| stm32mp131_133_135 LFBGA289 14x14
[IBIS ver]   4.2
[File name]   stm32mp131_133_135_lfbga289.ibs
[File Rev]   3.4
[Date]   06-03-2024
[Source]   Data Created at STMicroelectronics
[Disclaimer]  This information is for modeling purpose only and is
   not guaranteed.
   The information is subject to change without notice.
[Copyright]   Copyright 2024 STMicroelectronics Inc.
|  You might uncomment [Merged Pins] sections if handeled by the simulation tool
[Component] stm32mp131_133_135_lfbga289
[Manufacturer] STMicroelectronics
[Package]
| variable   typ   min   max
R_pkg  0  NA  NA
L_pkg  0  NA  NA
C_pkg  0  NA  NA
[Pin]   signal_name   model_name
T14  BYPASS_REG1V8  nc
G16  DDR_A0  PDDRIO_PAD
K15  DDR_A1  PDDRIO_PAD
J14  DDR_A10  PDDRIO_PAD
K13  DDR_A11  PDDRIO_PAD
K17  DDR_A12  PDDRIO_PAD
F14  DDR_A13  PDDRIO_PAD
L17  DDR_A14  PDDRIO_PAD
K16  DDR_A15  PDDRIO_PAD
F17  DDR_A2  PDDRIO_PAD
G15  DDR_A3  PDDRIO_PAD
M14  DDR_A4  PDDRIO_PAD
E16  DDR_A5  PDDRIO_PAD
M17  DDR_A6  PDDRIO_PAD
G14  DDR_A7  PDDRIO_PAD
L15  DDR_A8  PDDRIO_PAD
F16  DDR_A9  PDDRIO_PAD
L13  DDR_ATO  nc
G17  DDR_BA0  PDDRIO_PAD
L16  DDR_BA1  PDDRIO_PAD
G13  DDR_BA2  PDDRIO_PAD
J15  DDR_CASN  PDDRIO_PAD
K14  DDR_CKE  PDDRIO_PAD
J17  DDR_CLKN  PDDRIO_PAD
J16  DDR_CLKP  PDDRIO_PAD
H16  DDR_CSN  PDDRIO_PAD
B17  DDR_DQ0  PDDRIO_PAD
C15  DDR_DQ1  PDDRIO_PAD
N15  DDR_DQ10  PDDRIO_PAD
P15  DDR_DQ11  PDDRIO_PAD
R15  DDR_DQ12  PDDRIO_PAD
P16  DDR_DQ13  PDDRIO_PAD
T17  DDR_DQ14  PDDRIO_PAD
T16  DDR_DQ15  PDDRIO_PAD
E13  DDR_DQ2  PDDRIO_PAD
D17  DDR_DQ3  PDDRIO_PAD
B16  DDR_DQ4  PDDRIO_PAD
D16  DDR_DQ5  PDDRIO_PAD
E14  DDR_DQ6  PDDRIO_PAD
E15  DDR_DQ7  PDDRIO_PAD
N16  DDR_DQ8  PDDRIO_PAD
P17  DDR_DQ9  PDDRIO_PAD
D15  DDR_DQM0  PDDRIO_PAD
N14  DDR_DQM1  PDDRIO_PAD
C16  DDR_DQS0N  PDIFF_PAD
C17  DDR_DQS0P  PDIFF_PAD
R16  DDR_DQS1N  PDIFF_PAD
R17  DDR_DQS1P  PDIFF_PAD
L14  DDR_DTO0  PDDRIO_PAD
M16  DDR_DTO1  PDDRIO_PAD
H15  DDR_ODT  PDDRIO_PAD
H17  DDR_RASN  PDDRIO_PAD
E17  DDR_RESETN  PDDRIO_PAD
M13  DDR_VREF  nc
H13  DDR_WEN  PDDRIO_PAD
N17  DDR_ZQ  nc
N9  NJTRST  io8_ft
U10  NRST  nc
R9  NRST_CORE  nc
U3  PA0  io8_ft
R4  PA1  io8_ft
U15  PA10  io8usb_id_otg20_ft
T2  PA11  io8_ft_i2c
E3  PA12  io8_ft_hslv
P3  PA13  io8_ft
T12  PA14  io8_ft
E6  PA15  io8_ft_hslv
P5  PA2  io8_ft
N8  PA3  io8_ft_hslv
U5  PA4  io8_ft
U4  PA5  io8_ft
T8  PA6  io8_ft_hslv
U2  PA7  io8_ft_hslv
M2  PA8  io8_ft_i2c_hslv
A2  PA9  io8_ft_hslv
U7  PB0  io8_ft
T7  PB1  io8_ft_hslv
D10  PB10  io8_ft_hslv
N5  PB11  io8_ft_hslv_et
D9  PB12  io8_ft_hslv
E10  PB13  io8_ft_i2c_hslv
A13  PB14  io8_ft_hslv
B12  PB15  io8_ft_hslv
H4  PB2  io8_ft_hslv
C11  PB3  io8_ft_hslv
B13  PB4  io8_ft_hslv
C10  PB5  io8_ft_hslv
C1  PB6  io8_ft_hslv
A4  PB7  io8_ft_i2c
D1  PB8  io8_ft_i2c
A12  PB9  io8_ft_i2c_hslv
T3  PC0  io8_ft_hslv
U8  PC1  io8_ft_hslv_et
B14  PC10  io8_ft_i2c_hslv
C14  PC11  io8_ft_i2c_hslv
B15  PC12  io8_ft_hslv
K4  PC13  io8_ft
K1  PC14  io8_ft
K2  PC15  io8_ft
U9  PC2  io8_ft_hslv_et
T5  PC3  io8_ft_hslv
U6  PC4  io8_ft
R7  PC5  io8_ft
B11  PC6  io8_ft_hslv
A11  PC7  io8_ft_hslv
D14  PC8  io8_ft_hslv
A16  PC9  io8_ft_hslv
E4  PD0  io8_ft
D5  PD1  io8_ft_i2c_hslv
A3  PD10  io8_ft_hslv
E2  PD11  io8_ft_hslv
C6  PD12  io8_ft_i2c
J1  PD13  io8_ft_hslv
B3  PD14  io8_ft_i2c_hslv
C7  PD15  io8_ft_hslv
A15  PD2  io8_ft_hslv
B1  PD3  io8_ft_i2c
E7  PD4  io8_ft_hslv
A6  PD5  io8_ft_hslv
D2  PD6  io8_ft
N3  PD7  io8_ft_i2c_hslv
C5  PD8  io8_ft
E8  PD9  io8_ft_hslv
T10  PDR_ON  nc
D6  PE0  io8_ft_hslv
B5  PE1  io8_ft_hslv
B8  PE10  io8_ft
D4  PE11  io8_ft_hslv_et
B4  PE12  io8_ft_hslv
C4  PE13  io8_ft_i2c_hslv
C3  PE14  io8_ft_hslv
D8  PE15  io8_ft_i2c_hslv
L1  PE2  io8_ft_i2c_hslv
D13  PE3  io8_ft_hslv
H5  PE4  io8_ft_hslv
T9  PE5  io8_ft_hslv_et
N1  PE6  io8_ft_hslv_et
A5  PE7  io8_ft_hslv
A7  PE8  io8_ft_i2c
B6  PE9  io8_ft_hslv
C13  PF0  io8_ft_hslv
B9  PF1  io8_ft_i2c_hslv
G3  PF10  io8_ft_hslv
T6  PF11  io8_ft
T4  PF12  io8_ft_hslv_et
N6  PF13  io8_ft
P4  PF14  io8_ft
R10  PF15  io8_ft
E9  PF2  io8_ft_i2c_hslv
B10  PF3  io8_ft_i2c_hslv
L2  PF4  io8_ft_hslv
B2  PF5  io8_ft_hslv
G2  PF6  io8_ft_hslv_et
M1  PF7  io8_ft_hslv_et
G5  PF8  io8_ft_hslv
G1  PF9  io8_ft_hslv
D7  PG0  io8_ft_hslv
N2  PG1  io8_ft_hslv_et
F1  PG10  io8_ft_hslv
M3  PG11  io8_ft_hslv_et
T1  PG12  io8_ft
P8  PG13  io8_ft_hslv_et
P9  PG14  io8_ft_hslv_et
G4  PG15  io8_ft_hslv
R1  PG2  io8_ft
L5  PG3  io8_ft_et_i2c_hslv
A8  PG4  io8_ft_hslv
F2  PG5  io8_ft_hslv
A14  PG6  io8_ft_hslv
C9  PG7  io8_ft_hslv
F3  PG8  io8_ft_hslv
E1  PG9  io8_ft_i2c
P1  PH0  io8_ft
P2  PH1  io8_ft
E11  PH10  io8_ft_hslv
H1  PH11  io8_ft_i2c_hslv
C2  PH12  io8_ft_i2c_hslv
A10  PH13  io8_ft_i2c_hslv
B7  PH14  io8_ft_i2c_hslv
F4  PH2  io8_ft_hslv
R2  PH3  io8_ft_i2c_hslv
T15  PH4  io8_ft
R14  PH5  io8_ft
L3  PH6  io8_ft_i2c_hslv
H3  PH7  io8_ft_i2c_hslv
F5  PH8  io8_ft_i2c_hslv
A9  PH9  io8_ft_hslv
L4  PI0  io8_ft
K5  PI1  io8_ft
J3  PI2  io8_ft
H2  PI3  io8_ft
U14  PI4  io8_ft
P12  PI5  io8_ft
R12  PI6  io8_ft
U16  PI7  io8usb_vbus_otg20_ft
R3  PWR_CPU_ON  io8_ft
N13  PWR_LP  io8_ft
P14  PWR_ON  io8_ft
U13  USB_DM1  nc
U11  USB_DM2  nc
T13  USB_DP1  nc
T11  USB_DP2  nc
U12  USB_RREF  nc
J2  VBAT  power
G6  VDD  power
K6  VDD  power
L6  VDD  power
M6  VDD  power
M7  VDD  power
M8  VDD  power
M9  VDD  power
M10  VDD  power
M4  VDD_ANA  power
H8  VDD_CORE  power
H9  VDD_CORE  power
H10  VDD_CORE  power
J8  VDD_CORE  power
J10  VDD_CORE  power
K8  VDD_CORE  power
K9  VDD_CORE  power
K10  VDD_CORE  power
J13  VDD_CORE-J13  power
F6  VDD_CPU  power
F8  VDD_CPU  power
F9  VDD_CPU  power
H6  VDD_CPU  power
J6  VDD_CPU  power
G12  VDD_DDR  power
H12  VDD_DDR  power
J12  VDD_DDR  power
K12  VDD_DDR  power
L12  VDD_DDR  power
M12  VDD_DDR  power
N12  VDD_DDR  power
E12  VDD_DDR-E12-F12  power
F12  VDD_DDR-E12-F12  power
J5  VDD_PLL  power
R13  VDD_PLL2  power
P10  VDD3V3_USBHS  power
P7  VDDA  power
N11  VDDA1V1_REG  power
R11  VDDA1V8_REG  power
F7  VDD-F7-F10-F11  power
F10  VDD-F7-F10-F11  power
F11  VDD-F7-F10-F11  power
M11  VDD-M11  power
C12  VDDSDMMC1  power
D11  VDDSDMMC2  power
P6  VREFN  gnd
R6  VREFP  power
A1  VSS  gnd
A17  VSS  gnd
C8  VSS  gnd
D3  VSS  gnd
D12  VSS  gnd
E5  VSS  gnd
F13  VSS  gnd
F15  VSS  gnd
G7  VSS  gnd
G8  VSS  gnd
G9  VSS  gnd
G10  VSS  gnd
G11  VSS  gnd
H7  VSS  gnd
H11  VSS  gnd
H14  VSS  gnd
J7  VSS  gnd
J9  VSS  gnd
J11  VSS  gnd
K3  VSS  gnd
K7  VSS  gnd
K11  VSS  gnd
L7  VSS  gnd
L8  VSS  gnd
L9  VSS  gnd
L10  VSS  gnd
L11  VSS  gnd
M15  VSS  gnd
N4  VSS  gnd
P11  VSS  gnd
R5  VSS  gnd
R8  VSS  gnd
U1  VSS  gnd
U17  VSS  gnd
M5  VSS_ANA  gnd
J4  VSS_PLL  gnd
P13  VSS_PLL2  gnd
N10  VSS_USBHS  gnd
N7  VSSA  gnd
[Package Model]   501-bga-14x14-289-210615
[Pin Mapping]   pulldown_ref   pullup_ref   | Comment
T14  nc  nc  | Depending on IO usage
| T14  nc  nc  | Depending on IO usage
G16  gnd  vddddr
K15  gnd  vddddr
J14  gnd  vddddr
K13  gnd  vddddr
K17  gnd  vddddr
F14  gnd  vddddr
L17  gnd  vddddr
K16  gnd  vddddr
F17  gnd  vddddr
G15  gnd  vddddr
M14  gnd  vddddr
E16  gnd  vddddr
M17  gnd  vddddr
G14  gnd  vddddr
L15  gnd  vddddr
F16  gnd  vddddr
L13  nc  nc
G17  gnd  vddddr
L16  gnd  vddddr
G13  gnd  vddddr
J15  gnd  vddddr
K14  gnd  vddddr
J17  gnd  vddddr
J16  gnd  vddddr
H16  gnd  vddddr
B17  gnd  vddddr
C15  gnd  vddddr
N15  gnd  vddddr
P15  gnd  vddddr
R15  gnd  vddddr
P16  gnd  vddddr
T17  gnd  vddddr
T16  gnd  vddddr
E13  gnd  vddddr
D17  gnd  vddddr
B16  gnd  vddddr
D16  gnd  vddddr
E14  gnd  vddddr
E15  gnd  vddddr
N16  gnd  vddddr
P17  gnd  vddddr
D15  gnd  vddddr
N14  gnd  vddddr
C16  gnd  vddddr
C17  gnd  vddddr
R16  gnd  vddddr
R17  gnd  vddddr
L14  gnd  vddddr
M16  gnd  vddddr
H15  gnd  vddddr
H17  gnd  vddddr
E17  gnd  vddddr
M13  nc  nc
H13  gnd  vddddr
N17  nc  nc
N9  gnd  vddio
U10  nc  nc
R9  nc  nc
U3  gnd  vddio
R4  gnd  vddio
U15  gnd  vddio
T2  gnd  vddio
E3  gnd  vddio
P3  gnd  vddio
T12  gnd  vddio
E6  gnd  vddio
P5  gnd  vddio
N8  gnd  vddio
U5  gnd  vddio
U4  gnd  vddio
T8  gnd  vddio
U2  gnd  vddio
M2  gnd  vddio
A2  gnd  vddio
U7  gnd  vddio
T7  gnd  vddio
D10  gnd  vddio
N5  gnd  vddio
D9  gnd  vddio
E10  gnd  vddio
A13  gnd  vdds2  | Depending on IO usage
| A13  gnd  vddio  | Depending on IO usage
B12  gnd  vdds2  | Depending on IO usage
| B12  gnd  vddio  | Depending on IO usage
H4  gnd  vddio
C11  gnd  vdds2  | Depending on IO usage
| C11  gnd  vddio  | Depending on IO usage
B13  gnd  vdds2  | Depending on IO usage
| B13  gnd  vddio  | Depending on IO usage
C10  gnd  vddio
C1  gnd  vddio
A4  gnd  vddio
D1  gnd  vddio
A12  gnd  vddio
T3  gnd  vddio
U8  gnd  vddio
B14  gnd  vdds1  | Depending on IO usage
| B14  gnd  vddio  | Depending on IO usage
C14  gnd  vdds1  | Depending on IO usage
| C14  gnd  vddio  | Depending on IO usage
B15  gnd  vdds1  | Depending on IO usage
| B15  gnd  vddio  | Depending on IO usage
K4  gnd  vddio  | Depending on IO usage
| K4  gnd  vbat  | Depending on IO usage
K1  gnd  vddio  | Depending on IO usage
| K1  gnd  vbat  | Depending on IO usage
K2  gnd  vddio  | Depending on IO usage
| K2  gnd  vbat  | Depending on IO usage
U9  gnd  vddio
T5  gnd  vddio
U6  gnd  vddio
R7  gnd  vddio
B11  gnd  vddio
A11  gnd  vddio
D14  gnd  vdds1  | Depending on IO usage
| D14  gnd  vddio  | Depending on IO usage
A16  gnd  vdds1  | Depending on IO usage
| A16  gnd  vddio  | Depending on IO usage
E4  gnd  vddio
D5  gnd  vddio
A3  gnd  vddio
E2  gnd  vddio
C6  gnd  vddio
J1  gnd  vddio
B3  gnd  vddio
C7  gnd  vddio
A15  gnd  vdds1  | Depending on IO usage
| A15  gnd  vddio  | Depending on IO usage
B1  gnd  vddio
E7  gnd  vddio
A6  gnd  vddio
D2  gnd  vddio
N3  gnd  vddio
C5  gnd  vddio
E8  gnd  vddio
T10  nc  nc
D6  gnd  vddio
B5  gnd  vddio
B8  gnd  vddio
D4  gnd  vddio
B4  gnd  vddio
C4  gnd  vddio
C3  gnd  vddio
D8  gnd  vddio
L1  gnd  vddio
D13  gnd  vdds2  | Depending on IO usage
| D13  gnd  vddio  | Depending on IO usage
H5  gnd  vddio
T9  gnd  vddio
N1  gnd  vddio
A5  gnd  vddio
A7  gnd  vddio
B6  gnd  vddio
C13  gnd  vddio
B9  gnd  vddio
G3  gnd  vddio
T6  gnd  vddio
T4  gnd  vddio
N6  gnd  vddio
P4  gnd  vddio
R10  gnd  vddio
E9  gnd  vddio
B10  gnd  vddio
L2  gnd  vddio
B2  gnd  vddio
G2  gnd  vddio
M1  gnd  vddio
G5  gnd  vddio
G1  gnd  vddio
D7  gnd  vddio
N2  gnd  vddio
F1  gnd  vddio
M3  gnd  vddio
T1  gnd  vddio
P8  gnd  vddio
P9  gnd  vddio
G4  gnd  vddio
R1  gnd  vddio
L5  gnd  vddio
A8  gnd  vddio
F2  gnd  vddio
A14  gnd  vdds2  | Depending on IO usage
| A14  gnd  vddio  | Depending on IO usage
C9  gnd  vddio
F3  gnd  vddio
E1  gnd  vddio
P1  gnd  vddio
P2  gnd  vddio
E11  gnd  vddio
H1  gnd  vddio
C2  gnd  vddio
A10  gnd  vddio
B7  gnd  vddio
F4  gnd  vddio
R2  gnd  vddio
T15  gnd  vddio
R14  gnd  vddio
L3  gnd  vddio
H3  gnd  vddio
F5  gnd  vddio
A9  gnd  vddio
L4  gnd  vddio
K5  gnd  vddio  | Depending on IO usage
| K5  gnd  vbat  | Depending on IO usage
J3  gnd  vddio  | Depending on IO usage
| J3  gnd  vbat  | Depending on IO usage
H2  gnd  vddio  | Depending on IO usage
| H2  gnd  vbat  | Depending on IO usage
U14  gnd  vddio
P12  gnd  vddio
R12  gnd  vddio
U16  gnd  vddio
R3  gnd  vddio
N13  gnd  vddio
P14  gnd  vddio
U13  nc  nc  | Depending on IO usage
| U13  nc  nc  | Depending on IO usage
U11  nc  nc  | Depending on IO usage
| U11  nc  nc  | Depending on IO usage
T13  nc  nc  | Depending on IO usage
| T13  nc  nc  | Depending on IO usage
T11  nc  nc  | Depending on IO usage
| T11  nc  nc  | Depending on IO usage
U12  nc  nc  | Depending on IO usage
| U12  nc  nc  | Depending on IO usage
J2  nc  vbat
G6  nc  vddio
K6  nc  vddio
L6  nc  vddio
M6  nc  vddio
M7  nc  vddio
M8  nc  vddio
M9  nc  vddio
M10  nc  vddio
M4  nc  vddana
H8  nc  vddio  | Depending on IO usage
| H8  nc  vbat  | Depending on IO usage
H9  nc  vddio  | Depending on IO usage
| H9  nc  vbat  | Depending on IO usage
H10  nc  vddio  | Depending on IO usage
| H10  nc  vbat  | Depending on IO usage
J8  nc  vddio  | Depending on IO usage
| J8  nc  vbat  | Depending on IO usage
J10  nc  vddio  | Depending on IO usage
| J10  nc  vbat  | Depending on IO usage
K8  nc  vddio  | Depending on IO usage
| K8  nc  vbat  | Depending on IO usage
K9  nc  vddio  | Depending on IO usage
| K9  nc  vbat  | Depending on IO usage
K10  nc  vddio  | Depending on IO usage
| K10  nc  vbat  | Depending on IO usage
J13  nc  vddcore  | Depending on IO usage
| J13  nc  vbat  | Depending on IO usage
F6  nc  vddcpu
F8  nc  vddcpu
F9  nc  vddcpu
H6  nc  vddcpu
J6  nc  vddcpu
G12  nc  vddddr
H12  nc  vddddr
J12  nc  vddddr
K12  nc  vddddr
L12  nc  vddddr
M12  nc  vddddr
N12  nc  vddddr
E12  nc  vddddr
F12  nc  vddddr
J5  nc  vddpll
R13  nc  vddpll2
P10  nc  vdd3v3usbhs
P7  nc  vdda
N11  nc  vdda1v1
R11  nc  vdda1v8
F7  nc  vddio
F10  nc  vddio
F11  nc  vddio
M11  nc  vddio
C12  nc  vdds1
D11  nc  vdds2
P6  gnd  nc
R6  nc  vddio
A1  gnd  nc
A17  gnd  nc
C8  gnd  nc
D3  gnd  nc
D12  gnd  nc
E5  gnd  nc
F13  gnd  nc
F15  gnd  nc
G7  gnd  nc
G8  gnd  nc
G9  gnd  nc
G10  gnd  nc
G11  gnd  nc
H7  gnd  nc
H11  gnd  nc
H14  gnd  nc
J7  gnd  nc
J9  gnd  nc
J11  gnd  nc
K3  gnd  nc
K7  gnd  nc
K11  gnd  nc
L7  gnd  nc
L8  gnd  nc
L9  gnd  nc
L10  gnd  nc
L11  gnd  nc
M15  gnd  nc
N4  gnd  nc
P11  gnd  nc
R5  gnd  nc
R8  gnd  nc
U1  gnd  nc
U17  gnd  nc
M5  gnd  nc
J4  gnd  nc
P13  gnd  nc
N10  gnd  nc
N7  gnd  nc
[Diff_pin]   inv_pin   vdiff   tdelay_typ   tdelay_min   tdelay_max
J16   J17   0.320V   0ns   NA   NA   |CK
C17   C16   0.320V   0ns   NA   NA   |DQS0
R17   R16   0.320V   0ns   NA   NA   |DQS1
[Model Selector] PDIFF_PAD
MSD_D3RF2_18   DDR2 MSD_D3R_PDIFF Z0=18-Ohm
MSD_D3RF2_40   DDR2 MSD_D3R_PDIFF Z0=40-Ohm
MSD_D3RF2_48   DDR2 MSD_D3R_PDIFF Z0=48-Ohm
MSD_D3RF2_ODT150   DDR2 MSD_D3R_PDIFF cell 150-Ohm ODT Receiver
MSD_D3RF2_ODT50   DDR2 MSD_D3R_PDIFF cell 50-Ohm ODT Receiver
MSD_D3RF2_ODT75   DDR2 MSD_D3R_PDIFF cell 75-Ohm ODT Receiver
MSD_D3RF2_ODTOFF   DDR2 MSD_D3R_PDIFF cell ODT off Receiver
MSD_D3RF3_34   DDR3 MSD_D3R_PDIFF cell  Z0=34-Ohm
MSD_D3RF3_40   DDR3 MSD_D3R_PDIFF cell  Z0=40-Ohm
MSD_D3RF3_48   DDR3 MSD_D3R_PDIFF cell  Z0=48-Ohm
MSD_D3RF3L_34   DDR3L MSD_D3R_PDIFF cell  Z0=34-Ohm
MSD_D3RF3L_40   DDR3L MSD_D3R_PDIFF cell  Z0=40-Ohm
MSD_D3RF3L_48   DDR3L MSD_D3R_PDIFF cell  Z0=48-Ohm
MSD_D3RF3L_ODT120   DDR3L MSD_D3R_PDIFF cell 120-Ohm ODT Receiver
MSD_D3RF3L_ODT40   DDR3L MSD_D3R_PDIFF cell 40-Ohm ODT Receiver
MSD_D3RF3L_ODT60   DDR3L MSD_D3R_PDIFF cell 60-Ohm ODT Receiver
MSD_D3RF3L_ODTOFF   DDR3L MSD_D3R_PDIFF cell ODT off Receiver
MSD_D3RF3_ODT120   DDR3 MSD_D3R_PDIFF cell 120-Ohm ODT Receiver
MSD_D3RF3_ODT40   DDR3 MSD_D3R_PDIFF cell 40-Ohm ODT Receiver
MSD_D3RF3_ODT60   DDR3 MSD_D3R_PDIFF cell 60-Ohm ODT Receiver
MSD_D3RF3_ODTOFF   DDR3 MSD_D3R_PDIFF cell ODT off Receiver
MSD_D3RFL2_34   LPDDR2 MSD_D3R_PDIFF cell  Z0=34-Ohm
MSD_D3RFL2_40   LPDDR2 MSD_D3R_PDIFF cell  Z0=40-Ohm
MSD_D3RFL2_48   LPDDR2 MSD_D3R_PDIFF cell  Z0=48-Ohm
MSD_D3RFL2_60   LPDDR2 MSD_D3R_PDIFF cell  Z0=60-Ohm
MSD_D3RFL2_80   LPDDR2 MSD_D3R_PDIFF cell  Z0=80-Ohm
MSD_D3RFL2_ODTOFF   LPDDR2 MSD_D3R_PDIFF cell ODT off Receiver
MSD_D3RFL_48   LPDDR MSD_D3R_PDIFF cell  Z0=48-Ohm
MSD_D3RFL_ODTOFF   LPDDR MSD_D3R_PDIFF cell ODT off Receiver
MSD_D3RF2_18_OPEN   DDR2 MSD_D3R_PDIFF_PDQSR Z0=18-Ohm
MSD_D3RF2_40_OPEN   DDR2 MSD_D3R_PDIFF_PDQSR Z0=40-Ohm
MSD_D3RF2_48_OPEN   DDR2 MSD_D3R_PDIFF_PDQSR Z0=48-Ohm
MSD_D3RF2_18_PD344   DDR2 MSD_D3R_PDIFF_PDQSR Z0=18-Ohm
MSD_D3RF2_40_PD344   DDR2 MSD_D3R_PDIFF_PDQSR Z0=40-Ohm
MSD_D3RF2_48_PD344   DDR2 MSD_D3R_PDIFF_PDQSR Z0=48-Ohm
MSD_D3RF2_18_PD393   DDR2 MSD_D3R_PDIFF_PDQSR Z0=18-Ohm
MSD_D3RF2_40_PD393   DDR2 MSD_D3R_PDIFF_PDQSR Z0=40-Ohm
MSD_D3RF2_48_PD393   DDR2 MSD_D3R_PDIFF_PDQSR Z0=48-Ohm
MSD_D3RF2_18_PD458   DDR2 MSD_D3R_PDIFF_PDQSR Z0=18-Ohm
MSD_D3RF2_40_PD458   DDR2 MSD_D3R_PDIFF_PDQSR Z0=40-Ohm
MSD_D3RF2_48_PD458   DDR2 MSD_D3R_PDIFF_PDQSR Z0=48-Ohm
MSD_D3RF2_18_PD500   DDR2 MSD_D3R_PDIFF_PDQSR Z0=18-Ohm
MSD_D3RF2_40_PD500   DDR2 MSD_D3R_PDIFF_PDQSR Z0=40-Ohm
MSD_D3RF2_48_PD500   DDR2 MSD_D3R_PDIFF_PDQSR Z0=48-Ohm
MSD_D3RF2_18_PD550   DDR2 MSD_D3R_PDIFF_PDQSR Z0=18-Ohm
MSD_D3RF2_40_PD550   DDR2 MSD_D3R_PDIFF_PDQSR Z0=40-Ohm
MSD_D3RF2_48_PD550   DDR2 MSD_D3R_PDIFF_PDQSR Z0=48-Ohm
MSD_D3RF2_18_PD611   DDR2 MSD_D3R_PDIFF_PDQSR Z0=18-Ohm
MSD_D3RF2_40_PD611   DDR2 MSD_D3R_PDIFF_PDQSR Z0=40-Ohm
MSD_D3RF2_48_PD611   DDR2 MSD_D3R_PDIFF_PDQSR Z0=48-Ohm
MSD_D3RF2_18_PD688   DDR2 MSD_D3R_PDIFF_PDQSR Z0=18-Ohm
MSD_D3RF2_40_PD688   DDR2 MSD_D3R_PDIFF_PDQSR Z0=40-Ohm
MSD_D3RF2_48_PD688   DDR2 MSD_D3R_PDIFF_PDQSR Z0=48-Ohm
MSD_D3RF2_18_PU344   DDR2 MSD_D3R_PDIFF_PDQSR Z0=18-Ohm
MSD_D3RF2_40_PU344   DDR2 MSD_D3R_PDIFF_PDQSR Z0=40-Ohm
MSD_D3RF2_48_PU344   DDR2 MSD_D3R_PDIFF_PDQSR Z0=48-Ohm
MSD_D3RF2_18_PU393   DDR2 MSD_D3R_PDIFF_PDQSR Z0=18-Ohm
MSD_D3RF2_40_PU393   DDR2 MSD_D3R_PDIFF_PDQSR Z0=40-Ohm
MSD_D3RF2_48_PU393   DDR2 MSD_D3R_PDIFF_PDQSR Z0=48-Ohm
MSD_D3RF2_18_PU458   DDR2 MSD_D3R_PDIFF_PDQSR Z0=18-Ohm
MSD_D3RF2_40_PU458   DDR2 MSD_D3R_PDIFF_PDQSR Z0=40-Ohm
MSD_D3RF2_48_PU458   DDR2 MSD_D3R_PDIFF_PDQSR Z0=48-Ohm
MSD_D3RF2_18_PU500   DDR2 MSD_D3R_PDIFF_PDQSR Z0=18-Ohm
MSD_D3RF2_40_PU500   DDR2 MSD_D3R_PDIFF_PDQSR Z0=40-Ohm
MSD_D3RF2_48_PU500   DDR2 MSD_D3R_PDIFF_PDQSR Z0=48-Ohm
MSD_D3RF2_18_PU550   DDR2 MSD_D3R_PDIFF_PDQSR Z0=18-Ohm
MSD_D3RF2_40_PU550   DDR2 MSD_D3R_PDIFF_PDQSR Z0=40-Ohm
MSD_D3RF2_48_PU550   DDR2 MSD_D3R_PDIFF_PDQSR Z0=48-Ohm
MSD_D3RF2_18_PU611   DDR2 MSD_D3R_PDIFF_PDQSR Z0=18-Ohm
MSD_D3RF2_40_PU611   DDR2 MSD_D3R_PDIFF_PDQSR Z0=40-Ohm
MSD_D3RF2_48_PU611   DDR2 MSD_D3R_PDIFF_PDQSR Z0=48-Ohm
MSD_D3RF2_18_PU688   DDR2 MSD_D3R_PDIFF_PDQSR Z0=18-Ohm
MSD_D3RF2_40_PU688   DDR2 MSD_D3R_PDIFF_PDQSR Z0=40-Ohm
MSD_D3RF2_48_PU688   DDR2 MSD_D3R_PDIFF_PDQSR Z0=48-Ohm
MSD_D3RF2_18_PWRDWN   DDR2 MSD_D3R_PDIFF_PDQSR Z0=18-Ohm
MSD_D3RF2_40_PWRDWN   DDR2 MSD_D3R_PDIFF_PDQSR Z0=40-Ohm
MSD_D3RF2_48_PWRDWN   DDR2 MSD_D3R_PDIFF_PDQSR Z0=48-Ohm
MSD_D3RF3_34_OPEN   DDR3 MSD_D3R_PDIFF_PDQSR cell  Z0=34-Ohm
MSD_D3RF3_40_OPEN   DDR3 MSD_D3R_PDIFF_PDQSR cell  Z0=40-Ohm
MSD_D3RF3_48_OPEN   DDR3 MSD_D3R_PDIFF_PDQSR cell  Z0=48-Ohm
MSD_D3RF3_34_PD344   DDR3 MSD_D3R_PDIFF_PDQSR cell  Z0=34-Ohm
MSD_D3RF3_40_PD344   DDR3 MSD_D3R_PDIFF_PDQSR cell  Z0=40-Ohm
MSD_D3RF3_48_PD344   DDR3 MSD_D3R_PDIFF_PDQSR cell  Z0=48-Ohm
MSD_D3RF3_34_PD393   DDR3 MSD_D3R_PDIFF_PDQSR cell  Z0=34-Ohm
MSD_D3RF3_40_PD393   DDR3 MSD_D3R_PDIFF_PDQSR cell  Z0=40-Ohm
MSD_D3RF3_48_PD393   DDR3 MSD_D3R_PDIFF_PDQSR cell  Z0=48-Ohm
MSD_D3RF3_34_PD458   DDR3 MSD_D3R_PDIFF_PDQSR cell  Z0=34-Ohm
MSD_D3RF3_40_PD458   DDR3 MSD_D3R_PDIFF_PDQSR cell  Z0=40-Ohm
MSD_D3RF3_48_PD458   DDR3 MSD_D3R_PDIFF_PDQSR cell  Z0=48-Ohm
MSD_D3RF3_34_PD500   DDR3 MSD_D3R_PDIFF_PDQSR cell  Z0=34-Ohm
MSD_D3RF3_40_PD500   DDR3 MSD_D3R_PDIFF_PDQSR cell  Z0=40-Ohm
MSD_D3RF3_48_PD500   DDR3 MSD_D3R_PDIFF_PDQSR cell  Z0=48-Ohm
MSD_D3RF3_34_PD550   DDR3 MSD_D3R_PDIFF_PDQSR cell  Z0=34-Ohm
MSD_D3RF3_40_PD550   DDR3 MSD_D3R_PDIFF_PDQSR cell  Z0=40-Ohm
MSD_D3RF3_48_PD550   DDR3 MSD_D3R_PDIFF_PDQSR cell  Z0=48-Ohm
MSD_D3RF3_34_PD611   DDR3 MSD_D3R_PDIFF_PDQSR cell  Z0=34-Ohm
MSD_D3RF3_40_PD611   DDR3 MSD_D3R_PDIFF_PDQSR cell  Z0=40-Ohm
MSD_D3RF3_48_PD611   DDR3 MSD_D3R_PDIFF_PDQSR cell  Z0=48-Ohm
MSD_D3RF3_34_PD688   DDR3 MSD_D3R_PDIFF_PDQSR cell  Z0=34-Ohm
MSD_D3RF3_40_PD688   DDR3 MSD_D3R_PDIFF_PDQSR cell  Z0=40-Ohm
MSD_D3RF3_48_PD688   DDR3 MSD_D3R_PDIFF_PDQSR cell  Z0=48-Ohm
MSD_D3RF3_34_PU344   DDR3 MSD_D3R_PDIFF_PDQSR cell  Z0=34-Ohm
MSD_D3RF3_40_PU344   DDR3 MSD_D3R_PDIFF_PDQSR cell  Z0=40-Ohm
MSD_D3RF3_48_PU344   DDR3 MSD_D3R_PDIFF_PDQSR cell  Z0=48-Ohm
MSD_D3RF3_34_PU393   DDR3 MSD_D3R_PDIFF_PDQSR cell  Z0=34-Ohm
MSD_D3RF3_40_PU393   DDR3 MSD_D3R_PDIFF_PDQSR cell  Z0=40-Ohm
MSD_D3RF3_48_PU393   DDR3 MSD_D3R_PDIFF_PDQSR cell  Z0=48-Ohm
MSD_D3RF3_34_PU458   DDR3 MSD_D3R_PDIFF_PDQSR cell  Z0=34-Ohm
MSD_D3RF3_40_PU458   DDR3 MSD_D3R_PDIFF_PDQSR cell  Z0=40-Ohm
MSD_D3RF3_48_PU458   DDR3 MSD_D3R_PDIFF_PDQSR cell  Z0=48-Ohm
MSD_D3RF3_34_PU500   DDR3 MSD_D3R_PDIFF_PDQSR cell  Z0=34-Ohm
MSD_D3RF3_40_PU500   DDR3 MSD_D3R_PDIFF_PDQSR cell  Z0=40-Ohm
MSD_D3RF3_48_PU500   DDR3 MSD_D3R_PDIFF_PDQSR cell  Z0=48-Ohm
MSD_D3RF3_34_PU550   DDR3 MSD_D3R_PDIFF_PDQSR cell  Z0=34-Ohm
MSD_D3RF3_40_PU550   DDR3 MSD_D3R_PDIFF_PDQSR cell  Z0=40-Ohm
MSD_D3RF3_48_PU550   DDR3 MSD_D3R_PDIFF_PDQSR cell  Z0=48-Ohm
MSD_D3RF3_34_PU611   DDR3 MSD_D3R_PDIFF_PDQSR cell  Z0=34-Ohm
MSD_D3RF3_40_PU611   DDR3 MSD_D3R_PDIFF_PDQSR cell  Z0=40-Ohm
MSD_D3RF3_48_PU611   DDR3 MSD_D3R_PDIFF_PDQSR cell  Z0=48-Ohm
MSD_D3RF3_34_PU688   DDR3 MSD_D3R_PDIFF_PDQSR cell  Z0=34-Ohm
MSD_D3RF3_40_PU688   DDR3 MSD_D3R_PDIFF_PDQSR cell  Z0=40-Ohm
MSD_D3RF3_48_PU688   DDR3 MSD_D3R_PDIFF_PDQSR cell  Z0=48-Ohm
MSD_D3RF3_34_PWRDWN   DDR3 MSD_D3R_PDIFF_PDQSR cell  Z0=34-Ohm
MSD_D3RF3_40_PWRDWN   DDR3 MSD_D3R_PDIFF_PDQSR cell  Z0=40-Ohm
MSD_D3RF3_48_PWRDWN   DDR3 MSD_D3R_PDIFF_PDQSR cell  Z0=48-Ohm
MSD_D3RF3L_34_OPEN   DDR3L MSD_D3R_PDIFF_PDQSR cell  Z0=34-Ohm
MSD_D3RF3L_40_OPEN   DDR3L MSD_D3R_PDIFF_PDQSR cell  Z0=40-Ohm
MSD_D3RF3L_48_OPEN   DDR3L MSD_D3R_PDIFF_PDQSR cell  Z0=48-Ohm
MSD_D3RF3L_34_PD344   DDR3L MSD_D3R_PDIFF_PDQSR cell  Z0=34-Ohm
MSD_D3RF3L_40_PD344   DDR3L MSD_D3R_PDIFF_PDQSR cell  Z0=40-Ohm
MSD_D3RF3L_48_PD344   DDR3L MSD_D3R_PDIFF_PDQSR cell  Z0=48-Ohm
MSD_D3RF3L_34_PD393   DDR3L MSD_D3R_PDIFF_PDQSR cell  Z0=34-Ohm
MSD_D3RF3L_40_PD393   DDR3L MSD_D3R_PDIFF_PDQSR cell  Z0=40-Ohm
MSD_D3RF3L_48_PD393   DDR3L MSD_D3R_PDIFF_PDQSR cell  Z0=48-Ohm
MSD_D3RF3L_34_PD458   DDR3L MSD_D3R_PDIFF_PDQSR cell  Z0=34-Ohm
MSD_D3RF3L_40_PD458   DDR3L MSD_D3R_PDIFF_PDQSR cell  Z0=40-Ohm
MSD_D3RF3L_48_PD458   DDR3L MSD_D3R_PDIFF_PDQSR cell  Z0=48-Ohm
MSD_D3RF3L_34_PD500   DDR3L MSD_D3R_PDIFF_PDQSR cell  Z0=34-Ohm
MSD_D3RF3L_40_PD500   DDR3L MSD_D3R_PDIFF_PDQSR cell  Z0=40-Ohm
MSD_D3RF3L_48_PD500   DDR3L MSD_D3R_PDIFF_PDQSR cell  Z0=48-Ohm
MSD_D3RF3L_34_PD550   DDR3L MSD_D3R_PDIFF_PDQSR cell  Z0=34-Ohm
MSD_D3RF3L_40_PD550   DDR3L MSD_D3R_PDIFF_PDQSR cell  Z0=40-Ohm
MSD_D3RF3L_48_PD550   DDR3L MSD_D3R_PDIFF_PDQSR cell  Z0=48-Ohm
MSD_D3RF3L_34_PD611   DDR3L MSD_D3R_PDIFF_PDQSR cell  Z0=34-Ohm
MSD_D3RF3L_40_PD611   DDR3L MSD_D3R_PDIFF_PDQSR cell  Z0=40-Ohm
MSD_D3RF3L_48_PD611   DDR3L MSD_D3R_PDIFF_PDQSR cell  Z0=48-Ohm
MSD_D3RF3L_34_PD688   DDR3L MSD_D3R_PDIFF_PDQSR cell  Z0=34-Ohm
MSD_D3RF3L_40_PD688   DDR3L MSD_D3R_PDIFF_PDQSR cell  Z0=40-Ohm
MSD_D3RF3L_48_PD688   DDR3L MSD_D3R_PDIFF_PDQSR cell  Z0=48-Ohm
MSD_D3RF3L_34_PU344   DDR3L MSD_D3R_PDIFF_PDQSR cell  Z0=34-Ohm
MSD_D3RF3L_40_PU344   DDR3L MSD_D3R_PDIFF_PDQSR cell  Z0=40-Ohm
MSD_D3RF3L_48_PU344   DDR3L MSD_D3R_PDIFF_PDQSR cell  Z0=48-Ohm
MSD_D3RF3L_34_PU393   DDR3L MSD_D3R_PDIFF_PDQSR cell  Z0=34-Ohm
MSD_D3RF3L_40_PU393   DDR3L MSD_D3R_PDIFF_PDQSR cell  Z0=40-Ohm
MSD_D3RF3L_48_PU393   DDR3L MSD_D3R_PDIFF_PDQSR cell  Z0=48-Ohm
MSD_D3RF3L_34_PU458   DDR3L MSD_D3R_PDIFF_PDQSR cell  Z0=34-Ohm
MSD_D3RF3L_40_PU458   DDR3L MSD_D3R_PDIFF_PDQSR cell  Z0=40-Ohm
MSD_D3RF3L_48_PU458   DDR3L MSD_D3R_PDIFF_PDQSR cell  Z0=48-Ohm
MSD_D3RF3L_34_PU500   DDR3L MSD_D3R_PDIFF_PDQSR cell  Z0=34-Ohm
MSD_D3RF3L_40_PU500   DDR3L MSD_D3R_PDIFF_PDQSR cell  Z0=40-Ohm
MSD_D3RF3L_48_PU500   DDR3L MSD_D3R_PDIFF_PDQSR cell  Z0=48-Ohm
MSD_D3RF3L_34_PU550   DDR3L MSD_D3R_PDIFF_PDQSR cell  Z0=34-Ohm
MSD_D3RF3L_40_PU550   DDR3L MSD_D3R_PDIFF_PDQSR cell  Z0=40-Ohm
MSD_D3RF3L_48_PU550   DDR3L MSD_D3R_PDIFF_PDQSR cell  Z0=48-Ohm
MSD_D3RF3L_34_PU611   DDR3L MSD_D3R_PDIFF_PDQSR cell  Z0=34-Ohm
MSD_D3RF3L_40_PU611   DDR3L MSD_D3R_PDIFF_PDQSR cell  Z0=40-Ohm
MSD_D3RF3L_48_PU611   DDR3L MSD_D3R_PDIFF_PDQSR cell  Z0=48-Ohm
MSD_D3RF3L_34_PU688   DDR3L MSD_D3R_PDIFF_PDQSR cell  Z0=34-Ohm
MSD_D3RF3L_40_PU688   DDR3L MSD_D3R_PDIFF_PDQSR cell  Z0=40-Ohm
MSD_D3RF3L_48_PU688   DDR3L MSD_D3R_PDIFF_PDQSR cell  Z0=48-Ohm
MSD_D3RF3L_34_PWRDWN   DDR3L MSD_D3R_PDIFF_PDQSR cell  Z0=34-Ohm
MSD_D3RF3L_40_PWRDWN   DDR3L MSD_D3R_PDIFF_PDQSR cell  Z0=40-Ohm
MSD_D3RF3L_48_PWRDWN   DDR3L MSD_D3R_PDIFF_PDQSR cell  Z0=48-Ohm
MSD_D3RFL2_34_OPEN   LPDDR2 MSD_D3R_PDIFF_PDQSR cell  Z0=34-Ohm
MSD_D3RFL2_40_OPEN   LPDDR2 MSD_D3R_PDIFF_PDQSR cell  Z0=40-Ohm
MSD_D3RFL2_48_OPEN   LPDDR2 MSD_D3R_PDIFF_PDQSR cell  Z0=48-Ohm
MSD_D3RFL2_60_OPEN   LPDDR2 MSD_D3R_PDIFF_PDQSR cell  Z0=60-Ohm
MSD_D3RFL2_80_OPEN   LPDDR2 MSD_D3R_PDIFF_PDQSR cell  Z0=80-Ohm
MSD_D3RFL_48_OPEN   LPDDR MSD_D3R_PDIFF_PDQSR cell  Z0=48-Ohm
MSD_D3RFL2_34_PD344   LPDDR2 MSD_D3R_PDIFF_PDQSR cell  Z0=34-Ohm
MSD_D3RFL2_40_PD344   LPDDR2 MSD_D3R_PDIFF_PDQSR cell  Z0=40-Ohm
MSD_D3RFL2_48_PD344   LPDDR2 MSD_D3R_PDIFF_PDQSR cell  Z0=48-Ohm
MSD_D3RFL2_60_PD344   LPDDR2 MSD_D3R_PDIFF_PDQSR cell  Z0=60-Ohm
MSD_D3RFL2_80_PD344   LPDDR2 MSD_D3R_PDIFF_PDQSR cell  Z0=80-Ohm
MSD_D3RFL_48_PD344   LPDDR MSD_D3R_PDIFF_PDQSR cell  Z0=48-Ohm
MSD_D3RFL2_34_PD393   LPDDR2 MSD_D3R_PDIFF_PDQSR cell  Z0=34-Ohm
MSD_D3RFL2_40_PD393   LPDDR2 MSD_D3R_PDIFF_PDQSR cell  Z0=40-Ohm
MSD_D3RFL2_48_PD393   LPDDR2 MSD_D3R_PDIFF_PDQSR cell  Z0=48-Ohm
MSD_D3RFL2_60_PD393   LPDDR2 MSD_D3R_PDIFF_PDQSR cell  Z0=60-Ohm
MSD_D3RFL2_80_PD393   LPDDR2 MSD_D3R_PDIFF_PDQSR cell  Z0=80-Ohm
MSD_D3RFL_48_PD393   LPDDR MSD_D3R_PDIFF_PDQSR cell  Z0=48-Ohm
MSD_D3RFL2_34_PD458   LPDDR2 MSD_D3R_PDIFF_PDQSR cell  Z0=34-Ohm
MSD_D3RFL2_40_PD458   LPDDR2 MSD_D3R_PDIFF_PDQSR cell  Z0=40-Ohm
MSD_D3RFL2_48_PD458   LPDDR2 MSD_D3R_PDIFF_PDQSR cell  Z0=48-Ohm
MSD_D3RFL2_60_PD458   LPDDR2 MSD_D3R_PDIFF_PDQSR cell  Z0=60-Ohm
MSD_D3RFL2_80_PD458   LPDDR2 MSD_D3R_PDIFF_PDQSR cell  Z0=80-Ohm
MSD_D3RFL_48_PD458   LPDDR MSD_D3R_PDIFF_PDQSR cell  Z0=48-Ohm
MSD_D3RFL2_34_PD500   LPDDR2 MSD_D3R_PDIFF_PDQSR cell  Z0=34-Ohm
MSD_D3RFL2_40_PD500   LPDDR2 MSD_D3R_PDIFF_PDQSR cell  Z0=40-Ohm
MSD_D3RFL2_48_PD500   LPDDR2 MSD_D3R_PDIFF_PDQSR cell  Z0=48-Ohm
MSD_D3RFL2_60_PD500   LPDDR2 MSD_D3R_PDIFF_PDQSR cell  Z0=60-Ohm
MSD_D3RFL2_80_PD500   LPDDR2 MSD_D3R_PDIFF_PDQSR cell  Z0=80-Ohm
MSD_D3RFL_48_PD500   LPDDR MSD_D3R_PDIFF_PDQSR cell  Z0=48-Ohm
MSD_D3RFL2_34_PD550   LPDDR2 MSD_D3R_PDIFF_PDQSR cell  Z0=34-Ohm
MSD_D3RFL2_40_PD550   LPDDR2 MSD_D3R_PDIFF_PDQSR cell  Z0=40-Ohm
MSD_D3RFL2_48_PD550   LPDDR2 MSD_D3R_PDIFF_PDQSR cell  Z0=48-Ohm
MSD_D3RFL2_60_PD550   LPDDR2 MSD_D3R_PDIFF_PDQSR cell  Z0=60-Ohm
MSD_D3RFL2_80_PD550   LPDDR2 MSD_D3R_PDIFF_PDQSR cell  Z0=80-Ohm
MSD_D3RFL_48_PD550   LPDDR MSD_D3R_PDIFF_PDQSR cell  Z0=48-Ohm
MSD_D3RFL2_34_PD611   LPDDR2 MSD_D3R_PDIFF_PDQSR cell  Z0=34-Ohm
MSD_D3RFL2_40_PD611   LPDDR2 MSD_D3R_PDIFF_PDQSR cell  Z0=40-Ohm
MSD_D3RFL2_48_PD611   LPDDR2 MSD_D3R_PDIFF_PDQSR cell  Z0=48-Ohm
MSD_D3RFL2_60_PD611   LPDDR2 MSD_D3R_PDIFF_PDQSR cell  Z0=60-Ohm
MSD_D3RFL2_80_PD611   LPDDR2 MSD_D3R_PDIFF_PDQSR cell  Z0=80-Ohm
MSD_D3RFL_48_PD611   LPDDR MSD_D3R_PDIFF_PDQSR cell  Z0=48-Ohm
MSD_D3RFL2_34_PD688   LPDDR2 MSD_D3R_PDIFF_PDQSR cell  Z0=34-Ohm
MSD_D3RFL2_40_PD688   LPDDR2 MSD_D3R_PDIFF_PDQSR cell  Z0=40-Ohm
MSD_D3RFL2_48_PD688   LPDDR2 MSD_D3R_PDIFF_PDQSR cell  Z0=48-Ohm
MSD_D3RFL2_60_PD688   LPDDR2 MSD_D3R_PDIFF_PDQSR cell  Z0=60-Ohm
MSD_D3RFL2_80_PD688   LPDDR2 MSD_D3R_PDIFF_PDQSR cell  Z0=80-Ohm
MSD_D3RFL_48_PD688   LPDDR MSD_D3R_PDIFF_PDQSR cell  Z0=48-Ohm
MSD_D3RFL2_34_PU344   LPDDR2 MSD_D3R_PDIFF_PDQSR cell  Z0=34-Ohm
MSD_D3RFL2_40_PU344   LPDDR2 MSD_D3R_PDIFF_PDQSR cell  Z0=40-Ohm
MSD_D3RFL2_48_PU344   LPDDR2 MSD_D3R_PDIFF_PDQSR cell  Z0=48-Ohm
MSD_D3RFL2_60_PU344   LPDDR2 MSD_D3R_PDIFF_PDQSR cell  Z0=60-Ohm
MSD_D3RFL2_80_PU344   LPDDR2 MSD_D3R_PDIFF_PDQSR cell  Z0=80-Ohm
MSD_D3RFL_48_PU344   LPDDR MSD_D3R_PDIFF_PDQSR cell  Z0=48-Ohm
MSD_D3RFL2_34_PU393   LPDDR2 MSD_D3R_PDIFF_PDQSR cell  Z0=34-Ohm
MSD_D3RFL2_40_PU393   LPDDR2 MSD_D3R_PDIFF_PDQSR cell  Z0=40-Ohm
MSD_D3RFL2_48_PU393   LPDDR2 MSD_D3R_PDIFF_PDQSR cell  Z0=48-Ohm
MSD_D3RFL2_60_PU393   LPDDR2 MSD_D3R_PDIFF_PDQSR cell  Z0=60-Ohm
MSD_D3RFL2_80_PU393   LPDDR2 MSD_D3R_PDIFF_PDQSR cell  Z0=80-Ohm
MSD_D3RFL_48_PU393   LPDDR MSD_D3R_PDIFF_PDQSR cell  Z0=48-Ohm
MSD_D3RFL2_34_PU458   LPDDR2 MSD_D3R_PDIFF_PDQSR cell  Z0=34-Ohm
MSD_D3RFL2_40_PU458   LPDDR2 MSD_D3R_PDIFF_PDQSR cell  Z0=40-Ohm
MSD_D3RFL2_48_PU458   LPDDR2 MSD_D3R_PDIFF_PDQSR cell  Z0=48-Ohm
MSD_D3RFL2_60_PU458   LPDDR2 MSD_D3R_PDIFF_PDQSR cell  Z0=60-Ohm
MSD_D3RFL2_80_PU458   LPDDR2 MSD_D3R_PDIFF_PDQSR cell  Z0=80-Ohm
MSD_D3RFL_48_PU458   LPDDR MSD_D3R_PDIFF_PDQSR cell  Z0=48-Ohm
MSD_D3RFL2_34_PU500   LPDDR2 MSD_D3R_PDIFF_PDQSR cell  Z0=34-Ohm
MSD_D3RFL2_40_PU500   LPDDR2 MSD_D3R_PDIFF_PDQSR cell  Z0=40-Ohm
MSD_D3RFL2_48_PU500   LPDDR2 MSD_D3R_PDIFF_PDQSR cell  Z0=48-Ohm
MSD_D3RFL2_60_PU500   LPDDR2 MSD_D3R_PDIFF_PDQSR cell  Z0=60-Ohm
MSD_D3RFL2_80_PU500   LPDDR2 MSD_D3R_PDIFF_PDQSR cell  Z0=80-Ohm
MSD_D3RFL_48_PU500   LPDDR MSD_D3R_PDIFF_PDQSR cell  Z0=48-Ohm
MSD_D3RFL2_34_PU550   LPDDR2 MSD_D3R_PDIFF_PDQSR cell  Z0=34-Ohm
MSD_D3RFL2_40_PU550   LPDDR2 MSD_D3R_PDIFF_PDQSR cell  Z0=40-Ohm
MSD_D3RFL2_48_PU550   LPDDR2 MSD_D3R_PDIFF_PDQSR cell  Z0=48-Ohm
MSD_D3RFL2_60_PU550   LPDDR2 MSD_D3R_PDIFF_PDQSR cell  Z0=60-Ohm
MSD_D3RFL2_80_PU550   LPDDR2 MSD_D3R_PDIFF_PDQSR cell  Z0=80-Ohm
MSD_D3RFL_48_PU550   LPDDR MSD_D3R_PDIFF_PDQSR cell  Z0=48-Ohm
MSD_D3RFL2_34_PU611   LPDDR2 MSD_D3R_PDIFF_PDQSR cell  Z0=34-Ohm
MSD_D3RFL2_40_PU611   LPDDR2 MSD_D3R_PDIFF_PDQSR cell  Z0=40-Ohm
MSD_D3RFL2_48_PU611   LPDDR2 MSD_D3R_PDIFF_PDQSR cell  Z0=48-Ohm
MSD_D3RFL2_60_PU611   LPDDR2 MSD_D3R_PDIFF_PDQSR cell  Z0=60-Ohm
MSD_D3RFL2_80_PU611   LPDDR2 MSD_D3R_PDIFF_PDQSR cell  Z0=80-Ohm
MSD_D3RFL_48_PU611   LPDDR MSD_D3R_PDIFF_PDQSR cell  Z0=48-Ohm
MSD_D3RFL2_34_PU688   LPDDR2 MSD_D3R_PDIFF_PDQSR cell  Z0=34-Ohm
MSD_D3RFL2_40_PU688   LPDDR2 MSD_D3R_PDIFF_PDQSR cell  Z0=40-Ohm
MSD_D3RFL2_48_PU688   LPDDR2 MSD_D3R_PDIFF_PDQSR cell  Z0=48-Ohm
MSD_D3RFL2_60_PU688   LPDDR2 MSD_D3R_PDIFF_PDQSR cell  Z0=60-Ohm
MSD_D3RFL2_80_PU688   LPDDR2 MSD_D3R_PDIFF_PDQSR cell  Z0=80-Ohm
MSD_D3RFL_48_PU688   LPDDR MSD_D3R_PDIFF_PDQSR cell  Z0=48-Ohm
MSD_D3RFL2_34_PWRDWN   LPDDR2 MSD_D3R_PDIFF_PDQSR cell  Z0=34-Ohm
MSD_D3RFL2_40_PWRDWN   LPDDR2 MSD_D3R_PDIFF_PDQSR cell  Z0=40-Ohm
MSD_D3RFL2_48_PWRDWN   LPDDR2 MSD_D3R_PDIFF_PDQSR cell  Z0=48-Ohm
MSD_D3RFL2_60_PWRDWN   LPDDR2 MSD_D3R_PDIFF_PDQSR cell  Z0=60-Ohm
MSD_D3RFL2_80_PWRDWN   LPDDR2 MSD_D3R_PDIFF_PDQSR cell  Z0=80-Ohm
MSD_D3RFL_48_PWRDWN   LPDDR MSD_D3R_PDIFF_PDQSR cell  Z0=48-Ohm
MSD_D3RF2_ODT150_OPEN   DDR2 MSD_D3R_PDIFF_PDQSR cell 150-Ohm ODT Receiver
MSD_D3RF2_ODT50_OPEN   DDR2 MSD_D3R_PDIFF_PDQSR cell 50-Ohm ODT Receiver
MSD_D3RF2_ODT75_OPEN   DDR2 MSD_D3R_PDIFF_PDQSR cell 75-Ohm ODT Receiver
MSD_D3RF2_ODTOFF_OPEN   DDR2 MSD_D3R_PDIFF_PDQSR cell ODT off Receiver
MSD_D3RF2_ODT150_PD344   DDR2 MSD_D3R_PDIFF_PDQSR cell 150-Ohm ODT Receiver
MSD_D3RF2_ODT50_PD344   DDR2 MSD_D3R_PDIFF_PDQSR cell 50-Ohm ODT Receiver
MSD_D3RF2_ODT75_PD344   DDR2 MSD_D3R_PDIFF_PDQSR cell 75-Ohm ODT Receiver
MSD_D3RF2_ODTOFF_PD344   DDR2 MSD_D3R_PDIFF_PDQSR cell ODT off Receiver
MSD_D3RF2_ODT150_PD393   DDR2 MSD_D3R_PDIFF_PDQSR cell 150-Ohm ODT Receiver
MSD_D3RF2_ODT50_PD393   DDR2 MSD_D3R_PDIFF_PDQSR cell 50-Ohm ODT Receiver
MSD_D3RF2_ODT75_PD393   DDR2 MSD_D3R_PDIFF_PDQSR cell 75-Ohm ODT Receiver
MSD_D3RF2_ODTOFF_PD393   DDR2 MSD_D3R_PDIFF_PDQSR cell ODT off Receiver
MSD_D3RF2_ODT150_PD458   DDR2 MSD_D3R_PDIFF_PDQSR cell 150-Ohm ODT Receiver
MSD_D3RF2_ODT50_PD458   DDR2 MSD_D3R_PDIFF_PDQSR cell 50-Ohm ODT Receiver
MSD_D3RF2_ODT75_PD458   DDR2 MSD_D3R_PDIFF_PDQSR cell 75-Ohm ODT Receiver
MSD_D3RF2_ODTOFF_PD458   DDR2 MSD_D3R_PDIFF_PDQSR cell ODT off Receiver
MSD_D3RF2_ODT150_PD500   DDR2 MSD_D3R_PDIFF_PDQSR cell 150-Ohm ODT Receiver
MSD_D3RF2_ODT50_PD500   DDR2 MSD_D3R_PDIFF_PDQSR cell 50-Ohm ODT Receiver
MSD_D3RF2_ODT75_PD500   DDR2 MSD_D3R_PDIFF_PDQSR cell 75-Ohm ODT Receiver
MSD_D3RF2_ODTOFF_PD500   DDR2 MSD_D3R_PDIFF_PDQSR cell ODT off Receiver
MSD_D3RF2_ODT150_PD550   DDR2 MSD_D3R_PDIFF_PDQSR cell 150-Ohm ODT Receiver
MSD_D3RF2_ODT50_PD550   DDR2 MSD_D3R_PDIFF_PDQSR cell 50-Ohm ODT Receiver
MSD_D3RF2_ODT75_PD550   DDR2 MSD_D3R_PDIFF_PDQSR cell 75-Ohm ODT Receiver
MSD_D3RF2_ODTOFF_PD550   DDR2 MSD_D3R_PDIFF_PDQSR cell ODT off Receiver
MSD_D3RF2_ODT150_PD611   DDR2 MSD_D3R_PDIFF_PDQSR cell 150-Ohm ODT Receiver
MSD_D3RF2_ODT50_PD611   DDR2 MSD_D3R_PDIFF_PDQSR cell 50-Ohm ODT Receiver
MSD_D3RF2_ODT75_PD611   DDR2 MSD_D3R_PDIFF_PDQSR cell 75-Ohm ODT Receiver
MSD_D3RF2_ODTOFF_PD611   DDR2 MSD_D3R_PDIFF_PDQSR cell ODT off Receiver
MSD_D3RF2_ODT150_PD688   DDR2 MSD_D3R_PDIFF_PDQSR cell 150-Ohm ODT Receiver
MSD_D3RF2_ODT50_PD688   DDR2 MSD_D3R_PDIFF_PDQSR cell 50-Ohm ODT Receiver
MSD_D3RF2_ODT75_PD688   DDR2 MSD_D3R_PDIFF_PDQSR cell 75-Ohm ODT Receiver
MSD_D3RF2_ODTOFF_PD688   DDR2 MSD_D3R_PDIFF_PDQSR cell ODT off Receiver
MSD_D3RF2_ODT150_PU344   DDR2 MSD_D3R_PDIFF_PDQSR cell 150-Ohm ODT Receiver
MSD_D3RF2_ODT50_PU344   DDR2 MSD_D3R_PDIFF_PDQSR cell 50-Ohm ODT Receiver
MSD_D3RF2_ODT75_PU344   DDR2 MSD_D3R_PDIFF_PDQSR cell 75-Ohm ODT Receiver
MSD_D3RF2_ODTOFF_PU344   DDR2 MSD_D3R_PDIFF_PDQSR cell ODT off Receiver
MSD_D3RF2_ODT150_PU393   DDR2 MSD_D3R_PDIFF_PDQSR cell 150-Ohm ODT Receiver
MSD_D3RF2_ODT50_PU393   DDR2 MSD_D3R_PDIFF_PDQSR cell 50-Ohm ODT Receiver
MSD_D3RF2_ODT75_PU393   DDR2 MSD_D3R_PDIFF_PDQSR cell 75-Ohm ODT Receiver
MSD_D3RF2_ODTOFF_PU393   DDR2 MSD_D3R_PDIFF_PDQSR cell ODT off Receiver
MSD_D3RF2_ODT150_PU458   DDR2 MSD_D3R_PDIFF_PDQSR cell 150-Ohm ODT Receiver
MSD_D3RF2_ODT50_PU458   DDR2 MSD_D3R_PDIFF_PDQSR cell 50-Ohm ODT Receiver
MSD_D3RF2_ODT75_PU458   DDR2 MSD_D3R_PDIFF_PDQSR cell 75-Ohm ODT Receiver
MSD_D3RF2_ODTOFF_PU458   DDR2 MSD_D3R_PDIFF_PDQSR cell ODT off Receiver
MSD_D3RF2_ODT150_PU500   DDR2 MSD_D3R_PDIFF_PDQSR cell 150-Ohm ODT Receiver
MSD_D3RF2_ODT50_PU500   DDR2 MSD_D3R_PDIFF_PDQSR cell 50-Ohm ODT Receiver
MSD_D3RF2_ODT75_PU500   DDR2 MSD_D3R_PDIFF_PDQSR cell 75-Ohm ODT Receiver
MSD_D3RF2_ODTOFF_PU500   DDR2 MSD_D3R_PDIFF_PDQSR cell ODT off Receiver
MSD_D3RF2_ODT150_PU550   DDR2 MSD_D3R_PDIFF_PDQSR cell 150-Ohm ODT Receiver
MSD_D3RF2_ODT50_PU550   DDR2 MSD_D3R_PDIFF_PDQSR cell 50-Ohm ODT Receiver
MSD_D3RF2_ODT75_PU550   DDR2 MSD_D3R_PDIFF_PDQSR cell 75-Ohm ODT Receiver
MSD_D3RF2_ODTOFF_PU550   DDR2 MSD_D3R_PDIFF_PDQSR cell ODT off Receiver
MSD_D3RF2_ODT150_PU611   DDR2 MSD_D3R_PDIFF_PDQSR cell 150-Ohm ODT Receiver
MSD_D3RF2_ODT50_PU611   DDR2 MSD_D3R_PDIFF_PDQSR cell 50-Ohm ODT Receiver
MSD_D3RF2_ODT75_PU611   DDR2 MSD_D3R_PDIFF_PDQSR cell 75-Ohm ODT Receiver
MSD_D3RF2_ODTOFF_PU611   DDR2 MSD_D3R_PDIFF_PDQSR cell ODT off Receiver
MSD_D3RF2_ODT150_PU688   DDR2 MSD_D3R_PDIFF_PDQSR cell 150-Ohm ODT Receiver
MSD_D3RF2_ODT50_PU688   DDR2 MSD_D3R_PDIFF_PDQSR cell 50-Ohm ODT Receiver
MSD_D3RF2_ODT75_PU688   DDR2 MSD_D3R_PDIFF_PDQSR cell 75-Ohm ODT Receiver
MSD_D3RF2_ODTOFF_PU688   DDR2 MSD_D3R_PDIFF_PDQSR cell ODT off Receiver
MSD_D3RF2_ODT150_PWRDWN   DDR2 MSD_D3R_PDIFF_PDQSR cell 150-Ohm ODT Receiver
MSD_D3RF2_ODT50_PWRDWN   DDR2 MSD_D3R_PDIFF_PDQSR cell 50-Ohm ODT Receiver
MSD_D3RF2_ODT75_PWRDWN   DDR2 MSD_D3R_PDIFF_PDQSR cell 75-Ohm ODT Receiver
MSD_D3RF2_ODTOFF_PWRDWN   DDR2 MSD_D3R_PDIFF_PDQSR cell ODT off Receiver
MSD_D3RF3_ODT120_OPEN   DDR3 MSD_D3R_PDIFF_PDQSR cell 120-Ohm ODT Receiver
MSD_D3RF3_ODT40_OPEN   DDR3 MSD_D3R_PDIFF_PDQSR cell 40-Ohm ODT Receiver
MSD_D3RF3_ODT60_OPEN   DDR3 MSD_D3R_PDIFF_PDQSR cell 60-Ohm ODT Receiver
MSD_D3RF3_ODTOFF_OPEN   DDR3 MSD_D3R_PDIFF_PDQSR cell ODT off Receiver
MSD_D3RF3_ODT120_PD344   DDR3 MSD_D3R_PDIFF_PDQSR cell 120-Ohm ODT Receiver
MSD_D3RF3_ODT40_PD344   DDR3 MSD_D3R_PDIFF_PDQSR cell 40-Ohm ODT Receiver
MSD_D3RF3_ODT60_PD344   DDR3 MSD_D3R_PDIFF_PDQSR cell 60-Ohm ODT Receiver
MSD_D3RF3_ODTOFF_PD344   DDR3 MSD_D3R_PDIFF_PDQSR cell ODT off Receiver
MSD_D3RF3_ODT120_PD393   DDR3 MSD_D3R_PDIFF_PDQSR cell 120-Ohm ODT Receiver
MSD_D3RF3_ODT40_PD393   DDR3 MSD_D3R_PDIFF_PDQSR cell 40-Ohm ODT Receiver
MSD_D3RF3_ODT60_PD393   DDR3 MSD_D3R_PDIFF_PDQSR cell 60-Ohm ODT Receiver
MSD_D3RF3_ODTOFF_PD393   DDR3 MSD_D3R_PDIFF_PDQSR cell ODT off Receiver
MSD_D3RF3_ODT120_PD458   DDR3 MSD_D3R_PDIFF_PDQSR cell 120-Ohm ODT Receiver
MSD_D3RF3_ODT40_PD458   DDR3 MSD_D3R_PDIFF_PDQSR cell 40-Ohm ODT Receiver
MSD_D3RF3_ODT60_PD458   DDR3 MSD_D3R_PDIFF_PDQSR cell 60-Ohm ODT Receiver
MSD_D3RF3_ODTOFF_PD458   DDR3 MSD_D3R_PDIFF_PDQSR cell ODT off Receiver
MSD_D3RF3_ODT120_PD500   DDR3 MSD_D3R_PDIFF_PDQSR cell 120-Ohm ODT Receiver
MSD_D3RF3_ODT40_PD500   DDR3 MSD_D3R_PDIFF_PDQSR cell 40-Ohm ODT Receiver
MSD_D3RF3_ODT60_PD500   DDR3 MSD_D3R_PDIFF_PDQSR cell 60-Ohm ODT Receiver
MSD_D3RF3_ODTOFF_PD500   DDR3 MSD_D3R_PDIFF_PDQSR cell ODT off Receiver
MSD_D3RF3_ODT120_PD550   DDR3 MSD_D3R_PDIFF_PDQSR cell 120-Ohm ODT Receiver
MSD_D3RF3_ODT40_PD550   DDR3 MSD_D3R_PDIFF_PDQSR cell 40-Ohm ODT Receiver
MSD_D3RF3_ODT60_PD550   DDR3 MSD_D3R_PDIFF_PDQSR cell 60-Ohm ODT Receiver
MSD_D3RF3_ODTOFF_PD550   DDR3 MSD_D3R_PDIFF_PDQSR cell ODT off Receiver
MSD_D3RF3_ODT120_PD611   DDR3 MSD_D3R_PDIFF_PDQSR cell 120-Ohm ODT Receiver
MSD_D3RF3_ODT40_PD611   DDR3 MSD_D3R_PDIFF_PDQSR cell 40-Ohm ODT Receiver
MSD_D3RF3_ODT60_PD611   DDR3 MSD_D3R_PDIFF_PDQSR cell 60-Ohm ODT Receiver
MSD_D3RF3_ODTOFF_PD611   DDR3 MSD_D3R_PDIFF_PDQSR cell ODT off Receiver
MSD_D3RF3_ODT120_PD688   DDR3 MSD_D3R_PDIFF_PDQSR cell 120-Ohm ODT Receiver
MSD_D3RF3_ODT40_PD688   DDR3 MSD_D3R_PDIFF_PDQSR cell 40-Ohm ODT Receiver
MSD_D3RF3_ODT60_PD688   DDR3 MSD_D3R_PDIFF_PDQSR cell 60-Ohm ODT Receiver
MSD_D3RF3_ODTOFF_PD688   DDR3 MSD_D3R_PDIFF_PDQSR cell ODT off Receiver
MSD_D3RF3_ODT120_PU344   DDR3 MSD_D3R_PDIFF_PDQSR cell 120-Ohm ODT Receiver
MSD_D3RF3_ODT40_PU344   DDR3 MSD_D3R_PDIFF_PDQSR cell 40-Ohm ODT Receiver
MSD_D3RF3_ODT60_PU344   DDR3 MSD_D3R_PDIFF_PDQSR cell 60-Ohm ODT Receiver
MSD_D3RF3_ODTOFF_PU344   DDR3 MSD_D3R_PDIFF_PDQSR cell ODT off Receiver
MSD_D3RF3_ODT120_PU393   DDR3 MSD_D3R_PDIFF_PDQSR cell 120-Ohm ODT Receiver
MSD_D3RF3_ODT40_PU393   DDR3 MSD_D3R_PDIFF_PDQSR cell 40-Ohm ODT Receiver
MSD_D3RF3_ODT60_PU393   DDR3 MSD_D3R_PDIFF_PDQSR cell 60-Ohm ODT Receiver
MSD_D3RF3_ODTOFF_PU393   DDR3 MSD_D3R_PDIFF_PDQSR cell ODT off Receiver
MSD_D3RF3_ODT120_PU458   DDR3 MSD_D3R_PDIFF_PDQSR cell 120-Ohm ODT Receiver
MSD_D3RF3_ODT40_PU458   DDR3 MSD_D3R_PDIFF_PDQSR cell 40-Ohm ODT Receiver
MSD_D3RF3_ODT60_PU458   DDR3 MSD_D3R_PDIFF_PDQSR cell 60-Ohm ODT Receiver
MSD_D3RF3_ODTOFF_PU458   DDR3 MSD_D3R_PDIFF_PDQSR cell ODT off Receiver
MSD_D3RF3_ODT120_PU500   DDR3 MSD_D3R_PDIFF_PDQSR cell 120-Ohm ODT Receiver
MSD_D3RF3_ODT40_PU500   DDR3 MSD_D3R_PDIFF_PDQSR cell 40-Ohm ODT Receiver
MSD_D3RF3_ODT60_PU500   DDR3 MSD_D3R_PDIFF_PDQSR cell 60-Ohm ODT Receiver
MSD_D3RF3_ODTOFF_PU500   DDR3 MSD_D3R_PDIFF_PDQSR cell ODT off Receiver
MSD_D3RF3_ODT120_PU550   DDR3 MSD_D3R_PDIFF_PDQSR cell 120-Ohm ODT Receiver
MSD_D3RF3_ODT40_PU550   DDR3 MSD_D3R_PDIFF_PDQSR cell 40-Ohm ODT Receiver
MSD_D3RF3_ODT60_PU550   DDR3 MSD_D3R_PDIFF_PDQSR cell 60-Ohm ODT Receiver
MSD_D3RF3_ODTOFF_PU550   DDR3 MSD_D3R_PDIFF_PDQSR cell ODT off Receiver
MSD_D3RF3_ODT120_PU611   DDR3 MSD_D3R_PDIFF_PDQSR cell 120-Ohm ODT Receiver
MSD_D3RF3_ODT40_PU611   DDR3 MSD_D3R_PDIFF_PDQSR cell 40-Ohm ODT Receiver
MSD_D3RF3_ODT60_PU611   DDR3 MSD_D3R_PDIFF_PDQSR cell 60-Ohm ODT Receiver
MSD_D3RF3_ODTOFF_PU611   DDR3 MSD_D3R_PDIFF_PDQSR cell ODT off Receiver
MSD_D3RF3_ODT120_PU688   DDR3 MSD_D3R_PDIFF_PDQSR cell 120-Ohm ODT Receiver
MSD_D3RF3_ODT40_PU688   DDR3 MSD_D3R_PDIFF_PDQSR cell 40-Ohm ODT Receiver
MSD_D3RF3_ODT60_PU688   DDR3 MSD_D3R_PDIFF_PDQSR cell 60-Ohm ODT Receiver
MSD_D3RF3_ODTOFF_PU688   DDR3 MSD_D3R_PDIFF_PDQSR cell ODT off Receiver
MSD_D3RF3_ODT120_PWRDWN   DDR3 MSD_D3R_PDIFF_PDQSR cell 120-Ohm ODT Receiver
MSD_D3RF3_ODT40_PWRDWN   DDR3 MSD_D3R_PDIFF_PDQSR cell 40-Ohm ODT Receiver
MSD_D3RF3_ODT60_PWRDWN   DDR3 MSD_D3R_PDIFF_PDQSR cell 60-Ohm ODT Receiver
MSD_D3RF3_ODTOFF_PWRDWN   DDR3 MSD_D3R_PDIFF_PDQSR cell ODT off Receiver
MSD_D3RF3L_ODT120_OPEN   DDR3L MSD_D3R_PDIFF_PDQSR cell 120-Ohm ODT Receiver
MSD_D3RF3L_ODT40_OPEN   DDR3L MSD_D3R_PDIFF_PDQSR cell 40-Ohm ODT Receiver
MSD_D3RF3L_ODT60_OPEN   DDR3L MSD_D3R_PDIFF_PDQSR cell 60-Ohm ODT Receiver
MSD_D3RF3L_ODTOFF_OPEN   DDR3L MSD_D3R_PDIFF_PDQSR cell ODT off Receiver
MSD_D3RF3L_ODT120_PD344   DDR3L MSD_D3R_PDIFF_PDQSR cell 120-Ohm ODT Receiver
MSD_D3RF3L_ODT40_PD344   DDR3L MSD_D3R_PDIFF_PDQSR cell 40-Ohm ODT Receiver
MSD_D3RF3L_ODT60_PD344   DDR3L MSD_D3R_PDIFF_PDQSR cell 60-Ohm ODT Receiver
MSD_D3RF3L_ODTOFF_PD344   DDR3L MSD_D3R_PDIFF_PDQSR cell ODT off Receiver
MSD_D3RF3L_ODT120_PD393   DDR3L MSD_D3R_PDIFF_PDQSR cell 120-Ohm ODT Receiver
MSD_D3RF3L_ODT40_PD393   DDR3L MSD_D3R_PDIFF_PDQSR cell 40-Ohm ODT Receiver
MSD_D3RF3L_ODT60_PD393   DDR3L MSD_D3R_PDIFF_PDQSR cell 60-Ohm ODT Receiver
MSD_D3RF3L_ODTOFF_PD393   DDR3L MSD_D3R_PDIFF_PDQSR cell ODT off Receiver
MSD_D3RF3L_ODT120_PD458   DDR3L MSD_D3R_PDIFF_PDQSR cell 120-Ohm ODT Receiver
MSD_D3RF3L_ODT40_PD458   DDR3L MSD_D3R_PDIFF_PDQSR cell 40-Ohm ODT Receiver
MSD_D3RF3L_ODT60_PD458   DDR3L MSD_D3R_PDIFF_PDQSR cell 60-Ohm ODT Receiver
MSD_D3RF3L_ODTOFF_PD458   DDR3L MSD_D3R_PDIFF_PDQSR cell ODT off Receiver
MSD_D3RF3L_ODT120_PD500   DDR3L MSD_D3R_PDIFF_PDQSR cell 120-Ohm ODT Receiver
MSD_D3RF3L_ODT40_PD500   DDR3L MSD_D3R_PDIFF_PDQSR cell 40-Ohm ODT Receiver
MSD_D3RF3L_ODT60_PD500   DDR3L MSD_D3R_PDIFF_PDQSR cell 60-Ohm ODT Receiver
MSD_D3RF3L_ODTOFF_PD500   DDR3L MSD_D3R_PDIFF_PDQSR cell ODT off Receiver
MSD_D3RF3L_ODT120_PD550   DDR3L MSD_D3R_PDIFF_PDQSR cell 120-Ohm ODT Receiver
MSD_D3RF3L_ODT40_PD550   DDR3L MSD_D3R_PDIFF_PDQSR cell 40-Ohm ODT Receiver
MSD_D3RF3L_ODT60_PD550   DDR3L MSD_D3R_PDIFF_PDQSR cell 60-Ohm ODT Receiver
MSD_D3RF3L_ODTOFF_PD550   DDR3L MSD_D3R_PDIFF_PDQSR cell ODT off Receiver
MSD_D3RF3L_ODT120_PD611   DDR3L MSD_D3R_PDIFF_PDQSR cell 120-Ohm ODT Receiver
MSD_D3RF3L_ODT40_PD611   DDR3L MSD_D3R_PDIFF_PDQSR cell 40-Ohm ODT Receiver
MSD_D3RF3L_ODT60_PD611   DDR3L MSD_D3R_PDIFF_PDQSR cell 60-Ohm ODT Receiver
MSD_D3RF3L_ODTOFF_PD611   DDR3L MSD_D3R_PDIFF_PDQSR cell ODT off Receiver
MSD_D3RF3L_ODT120_PD688   DDR3L MSD_D3R_PDIFF_PDQSR cell 120-Ohm ODT Receiver
MSD_D3RF3L_ODT40_PD688   DDR3L MSD_D3R_PDIFF_PDQSR cell 40-Ohm ODT Receiver
MSD_D3RF3L_ODT60_PD688   DDR3L MSD_D3R_PDIFF_PDQSR cell 60-Ohm ODT Receiver
MSD_D3RF3L_ODTOFF_PD688   DDR3L MSD_D3R_PDIFF_PDQSR cell ODT off Receiver
MSD_D3RF3L_ODT120_PU344   DDR3L MSD_D3R_PDIFF_PDQSR cell 120-Ohm ODT Receiver
MSD_D3RF3L_ODT40_PU344   DDR3L MSD_D3R_PDIFF_PDQSR cell 40-Ohm ODT Receiver
MSD_D3RF3L_ODT60_PU344   DDR3L MSD_D3R_PDIFF_PDQSR cell 60-Ohm ODT Receiver
MSD_D3RF3L_ODTOFF_PU344   DDR3L MSD_D3R_PDIFF_PDQSR cell ODT off Receiver
MSD_D3RF3L_ODT120_PU393   DDR3L MSD_D3R_PDIFF_PDQSR cell 120-Ohm ODT Receiver
MSD_D3RF3L_ODT40_PU393   DDR3L MSD_D3R_PDIFF_PDQSR cell 40-Ohm ODT Receiver
MSD_D3RF3L_ODT60_PU393   DDR3L MSD_D3R_PDIFF_PDQSR cell 60-Ohm ODT Receiver
MSD_D3RF3L_ODTOFF_PU393   DDR3L MSD_D3R_PDIFF_PDQSR cell ODT off Receiver
MSD_D3RF3L_ODT120_PU458   DDR3L MSD_D3R_PDIFF_PDQSR cell 120-Ohm ODT Receiver
MSD_D3RF3L_ODT40_PU458   DDR3L MSD_D3R_PDIFF_PDQSR cell 40-Ohm ODT Receiver
MSD_D3RF3L_ODT60_PU458   DDR3L MSD_D3R_PDIFF_PDQSR cell 60-Ohm ODT Receiver
MSD_D3RF3L_ODTOFF_PU458   DDR3L MSD_D3R_PDIFF_PDQSR cell ODT off Receiver
MSD_D3RF3L_ODT120_PU500   DDR3L MSD_D3R_PDIFF_PDQSR cell 120-Ohm ODT Receiver
MSD_D3RF3L_ODT40_PU500   DDR3L MSD_D3R_PDIFF_PDQSR cell 40-Ohm ODT Receiver
MSD_D3RF3L_ODT60_PU500   DDR3L MSD_D3R_PDIFF_PDQSR cell 60-Ohm ODT Receiver
MSD_D3RF3L_ODTOFF_PU500   DDR3L MSD_D3R_PDIFF_PDQSR cell ODT off Receiver
MSD_D3RF3L_ODT120_PU550   DDR3L MSD_D3R_PDIFF_PDQSR cell 120-Ohm ODT Receiver
MSD_D3RF3L_ODT40_PU550   DDR3L MSD_D3R_PDIFF_PDQSR cell 40-Ohm ODT Receiver
MSD_D3RF3L_ODT60_PU550   DDR3L MSD_D3R_PDIFF_PDQSR cell 60-Ohm ODT Receiver
MSD_D3RF3L_ODTOFF_PU550   DDR3L MSD_D3R_PDIFF_PDQSR cell ODT off Receiver
MSD_D3RF3L_ODT120_PU611   DDR3L MSD_D3R_PDIFF_PDQSR cell 120-Ohm ODT Receiver
MSD_D3RF3L_ODT40_PU611   DDR3L MSD_D3R_PDIFF_PDQSR cell 40-Ohm ODT Receiver
MSD_D3RF3L_ODT60_PU611   DDR3L MSD_D3R_PDIFF_PDQSR cell 60-Ohm ODT Receiver
MSD_D3RF3L_ODTOFF_PU611   DDR3L MSD_D3R_PDIFF_PDQSR cell ODT off Receiver
MSD_D3RF3L_ODT120_PU688   DDR3L MSD_D3R_PDIFF_PDQSR cell 120-Ohm ODT Receiver
MSD_D3RF3L_ODT40_PU688   DDR3L MSD_D3R_PDIFF_PDQSR cell 40-Ohm ODT Receiver
MSD_D3RF3L_ODT60_PU688   DDR3L MSD_D3R_PDIFF_PDQSR cell 60-Ohm ODT Receiver
MSD_D3RF3L_ODTOFF_PU688   DDR3L MSD_D3R_PDIFF_PDQSR cell ODT off Receiver
MSD_D3RF3L_ODT120_PWRDWN   DDR3L MSD_D3R_PDIFF_PDQSR cell 120-Ohm ODT Receiver
MSD_D3RF3L_ODT40_PWRDWN   DDR3L MSD_D3R_PDIFF_PDQSR cell 40-Ohm ODT Receiver
MSD_D3RF3L_ODT60_PWRDWN   DDR3L MSD_D3R_PDIFF_PDQSR cell 60-Ohm ODT Receiver
MSD_D3RF3L_ODTOFF_PWRDWN   DDR3L MSD_D3R_PDIFF_PDQSR cell ODT off Receiver
MSD_D3RFL2_ODTOFF_OPEN   LPDDR2 MSD_D3R_PDIFF_PDQSR cell ODT off Receiver
MSD_D3RFL_ODTOFF_OPEN   LPDDR MSD_D3R_PDIFF_PDQSR cell ODT off Receiver
MSD_D3RFL2_ODTOFF_PD344   LPDDR2 MSD_D3R_PDIFF_PDQSR cell ODT off Receiver
MSD_D3RFL_ODTOFF_PD344   LPDDR MSD_D3R_PDIFF_PDQSR cell ODT off Receiver
MSD_D3RFL2_ODTOFF_PD393   LPDDR2 MSD_D3R_PDIFF_PDQSR cell ODT off Receiver
MSD_D3RFL_ODTOFF_PD393   LPDDR MSD_D3R_PDIFF_PDQSR cell ODT off Receiver
MSD_D3RFL2_ODTOFF_PD458   LPDDR2 MSD_D3R_PDIFF_PDQSR cell ODT off Receiver
MSD_D3RFL_ODTOFF_PD458   LPDDR MSD_D3R_PDIFF_PDQSR cell ODT off Receiver
MSD_D3RFL2_ODTOFF_PD500   LPDDR2 MSD_D3R_PDIFF_PDQSR cell ODT off Receiver
MSD_D3RFL_ODTOFF_PD500   LPDDR MSD_D3R_PDIFF_PDQSR cell ODT off Receiver
MSD_D3RFL2_ODTOFF_PD550   LPDDR2 MSD_D3R_PDIFF_PDQSR cell ODT off Receiver
MSD_D3RFL_ODTOFF_PD550   LPDDR MSD_D3R_PDIFF_PDQSR cell ODT off Receiver
MSD_D3RFL2_ODTOFF_PD611   LPDDR2 MSD_D3R_PDIFF_PDQSR cell ODT off Receiver
MSD_D3RFL_ODTOFF_PD611   LPDDR MSD_D3R_PDIFF_PDQSR cell ODT off Receiver
MSD_D3RFL2_ODTOFF_PD688   LPDDR2 MSD_D3R_PDIFF_PDQSR cell ODT off Receiver
MSD_D3RFL_ODTOFF_PD688   LPDDR MSD_D3R_PDIFF_PDQSR cell ODT off Receiver
MSD_D3RFL2_ODTOFF_PU344   LPDDR2 MSD_D3R_PDIFF_PDQSR cell ODT off Receiver
MSD_D3RFL_ODTOFF_PU344   LPDDR MSD_D3R_PDIFF_PDQSR cell ODT off Receiver
MSD_D3RFL2_ODTOFF_PU393   LPDDR2 MSD_D3R_PDIFF_PDQSR cell ODT off Receiver
MSD_D3RFL_ODTOFF_PU393   LPDDR MSD_D3R_PDIFF_PDQSR cell ODT off Receiver
MSD_D3RFL2_ODTOFF_PU458   LPDDR2 MSD_D3R_PDIFF_PDQSR cell ODT off Receiver
MSD_D3RFL_ODTOFF_PU458   LPDDR MSD_D3R_PDIFF_PDQSR cell ODT off Receiver
MSD_D3RFL2_ODTOFF_PU500   LPDDR2 MSD_D3R_PDIFF_PDQSR cell ODT off Receiver
MSD_D3RFL_ODTOFF_PU500   LPDDR MSD_D3R_PDIFF_PDQSR cell ODT off Receiver
MSD_D3RFL2_ODTOFF_PU550   LPDDR2 MSD_D3R_PDIFF_PDQSR cell ODT off Receiver
MSD_D3RFL_ODTOFF_PU550   LPDDR MSD_D3R_PDIFF_PDQSR cell ODT off Receiver
MSD_D3RFL2_ODTOFF_PU611   LPDDR2 MSD_D3R_PDIFF_PDQSR cell ODT off Receiver
MSD_D3RFL_ODTOFF_PU611   LPDDR MSD_D3R_PDIFF_PDQSR cell ODT off Receiver
MSD_D3RFL2_ODTOFF_PU688   LPDDR2 MSD_D3R_PDIFF_PDQSR cell ODT off Receiver
MSD_D3RFL_ODTOFF_PU688   LPDDR MSD_D3R_PDIFF_PDQSR cell ODT off Receiver
MSD_D3RFL2_ODTOFF_PWRDWN   LPDDR2 MSD_D3R_PDIFF_PDQSR cell ODT off Receiver
MSD_D3RFL_ODTOFF_PWRDWN   LPDDR MSD_D3R_PDIFF_PDQSR cell ODT off Receiver
[Model Selector] PDDRIO_PAD
MSD_D3RP2_18   DDR2 MSD_D3R_PDDRIO Z0=18-Ohm
MSD_D3RP2_40   DDR2 MSD_D3R_PDDRIO Z0=40-Ohm
MSD_D3RP2_48   DDR2 MSD_D3R_PDDRIO Z0=48-Ohm
MSD_D3RP2_ODT150   DDR2 MSD_D3R_PDDRIO cell 150-Ohm ODT Receiver
MSD_D3RP2_ODT50   DDR2 MSD_D3R_PDDRIO cell 50-Ohm ODT Receiver
MSD_D3RP2_ODT75   DDR2 MSD_D3R_PDDRIO cell 75-Ohm ODT Receiver
MSD_D3RP2_ODTOFF   DDR2 MSD_D3R_PDDRIO cell ODT off Receiver
MSD_D3RP3_34   DDR3 MSD_D3R_PDDRIO cell  Z0=34-Ohm
MSD_D3RP3_40   DDR3 MSD_D3R_PDDRIO cell  Z0=40-Ohm
MSD_D3RP3_48   DDR3 MSD_D3R_PDDRIO cell  Z0=48-Ohm
MSD_D3RP3L_34   DDR3L MSD_D3R_PDDRIO cell  Z0=34-Ohm
MSD_D3RP3L_40   DDR3L MSD_D3R_PDDRIO cell  Z0=40-Ohm
MSD_D3RP3L_48   DDR3L MSD_D3R_PDDRIO cell  Z0=48-Ohm
MSD_D3RP3L_ODT120   DDR3L MSD_D3R_PDDRIO cell 120-Ohm ODT Receiver
MSD_D3RP3L_ODT40   DDR3L MSD_D3R_PDDRIO cell 40-Ohm ODT Receiver
MSD_D3RP3L_ODT60   DDR3L MSD_D3R_PDDRIO cell 60-Ohm ODT Receiver
MSD_D3RP3L_ODTOFF   DDR3L MSD_D3R_PDDRIO cell ODT off Receiver
MSD_D3RP3_ODT120   DDR3 MSD_D3R_PDDRIO cell 120-Ohm ODT Receiver
MSD_D3RP3_ODT40   DDR3 MSD_D3R_PDDRIO cell 40-Ohm ODT Receiver
MSD_D3RP3_ODT60   DDR3 MSD_D3R_PDDRIO cell 60-Ohm ODT Receiver
MSD_D3RP3_ODTOFF   DDR3 MSD_D3R_PDDRIO cell ODT off Receiver
MSD_D3RPL2_34   LPDDR2 MSD_D3R_PDDRIO cell  Z0=34-Ohm
MSD_D3RPL2_40   LPDDR2 MSD_D3R_PDDRIO cell  Z0=40-Ohm
MSD_D3RPL2_48   LPDDR2 MSD_D3R_PDDRIO cell  Z0=48-Ohm
MSD_D3RPL2_60   LPDDR2 MSD_D3R_PDDRIO cell  Z0=60-Ohm
MSD_D3RPL2_80   LPDDR2 MSD_D3R_PDDRIO cell  Z0=80-Ohm
MSD_D3RPL2_ODTOFF   LPDDR2 MSD_D3R_PDDRIO cell ODT off Receiver
MSD_D3RPL_48   LPDDR MSD_D3R_PDDRIO cell  Z0=48-Ohm
MSD_D3RPL_ODTOFF   LPDDR MSD_D3R_PDDRIO cell ODT off Receiver
[Model Selector] io8_ft
io8_ft_ls_1v2   "GPIO - 5V tolerant - 1.2V range - Low speed"
io8_ft_ms_1v2   "GPIO - 5V tolerant - 1.2V range - Med speed"
io8_ft_hs_1v2   "GPIO - 5V tolerant - 1.2V range - High speed"
io8_ft_fs_1v2   "GPIO - 5V tolerant - 1.2V range - Fast speed"
io8_ft_hs_1v8   "GPIO - 5V tolerant - 1.8V range - High speed -"
io8_ft_fs_1v8   "GPIO - 5V tolerant - 1.8V range - Fast speed -"
io8_ft_ms_1v8   "GPIO - 5V tolerant - 1.8V range - Medium speed"
io8_ft_ls_1v8   "GPIO - 5V tolerant - 1.8V range - Low speed"
io8_ft_hs_3v3   "GPIO - 5V tolerant - 3.3V range - High speed"
io8_ft_fs_3v3   "GPIO - 5V tolerant - 3.3V range - Fast speed"
io8_ft_ms_3v3   "GPIO - 5V tolerant - 3.3V range - Medium speed"
io8_ft_ls_3v3   "GPIO - 5V tolerant - 3.3V range - Low speed"
[Model Selector] io8_ft_hslv
io8_ft_ls_1v2   "GPIO - 5V tolerant - 1.2V range - Low speed"
io8_ft_ms_1v2   "GPIO - 5V tolerant - 1.2V range - Med speed"
io8_ft_hs_1v2   "GPIO - 5V tolerant - 1.2V range - High speed"
io8_ft_fs_1v2   "GPIO - 5V tolerant - 1.2V range - Fast speed"
io8_ft_hs_1v8   "GPIO - 5V tolerant - 1.8V range - High speed -"
io8_ft_fs_1v8   "GPIO - 5V tolerant - 1.8V range - Fast speed -"
io8_ft_ms_1v8   "GPIO - 5V tolerant - 1.8V range - Medium speed"
io8_ft_ls_1v8   "GPIO - 5V tolerant - 1.8V range - Low speed"
io8_ft_hs_3v3   "GPIO - 5V tolerant - 3.3V range - High speed"
io8_ft_fs_3v3   "GPIO - 5V tolerant - 3.3V range - Fast speed"
io8_ft_ms_3v3   "GPIO - 5V tolerant - 3.3V range - Medium speed"
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| Models and submodels in the file (574): io8_ft_ls_1v2 (I/O), io8_ft_ms_1v2 (I/O), io8_ft_fs_1v2 (I/O), io8_ft_hs_1v2 (I/O), io8_ft_ls_1v8 (I/O), io8_ft_ms_1v8 (I/O), io8_ft_fs_1v8 (I/O), io8_ft_hs_1v8 (I/O), io8_ft_ls_3v3 (I/O), io8_ft_ms_3v3 (I/O), io8_ft_fs_3v3 (I/O), io8_ft_hs_3v3 (I/O), io8_ft_hslv_et_ls_1v2 (I/O), io8_ft_hslv_et_ms_1v2 (I/O), io8_ft_hslv_et_fs_1v2 (I/O), io8_ft_hslv_et_hs_1v2 (I/O), io8_ft_hslv_et_ls_1v8 (I/O), io8_ft_hslv_et_ms_1v8 (I/O), io8_ft_hslv_et_fs_1v8 (I/O), io8_ft_hslv_et_hs_1v8 (I/O), io8_ft_hslv_et_ls_2v5 (I/O), io8_ft_hslv_et_ms_2v5 (I/O), io8_ft_hslv_et_fs_2v5 (I/O), io8_ft_hslv_et_hs_2v5 (I/O), io8_ft_hslv_ls_1v2 (I/O), io8_ft_hslv_ms_1v2 (I/O), io8_ft_hslv_fs_1v2 (I/O), io8_ft_hslv_hs_1v2 (I/O), io8_ft_hslv_ls_1v8 (I/O), io8_ft_hslv_ms_1v8 (I/O), io8_ft_hslv_fs_1v8 (I/O), io8_ft_hslv_hs_1v8 (I/O), io8_ft_hslv_ls_2v5 (I/O), io8_ft_hslv_ms_2v5 (I/O), io8_ft_hslv_fs_2v5 (I/O), io8_ft_hslv_hs_2v5 (I/O), io8_ft_i2c_ls_1v2 (I/O_open_drain), io8_ft_i2c_ms_1v2 (I/O_open_drain), io8_ft_i2c_fs_1v2 (I/O_open_drain), io8_ft_i2c_hs_1v2 (I/O_open_drain), io8_ft_i2c_ls_1v8 (I/O_open_drain), io8_ft_i2c_ms_1v8 (I/O_open_drain), io8_ft_i2c_fs_1v8 (I/O_open_drain), io8_ft_i2c_hs_1v8 (I/O_open_drain), io8_ft_i2c_ls_3v3 (I/O_open_drain), io8_ft_i2c_ms_3v3 (I/O_open_drain), io8_ft_i2c_fs_3v3 (I/O_open_drain), io8_ft_i2c_hs_3v3 (I/O_open_drain), io8usb_adp_3v3 (I/O), io8usb_vbus_3v3 (I/O), io8usb_id_ft_nopup (Input), io8usb_id_ft_pup (Input), MSD_D3RF2_18 (I/O), MSD_D3RF2_40 (I/O), MSD_D3RF2_48 (I/O), MSD_D3RF2_ODT150 (Input), MSD_D3RF2_ODT50 (Input), MSD_D3RF2_ODT75 (Input), MSD_D3RF2_ODTOFF (Input), MSD_D3RF3_34 (I/O), MSD_D3RF3_40 (I/O), MSD_D3RF3_48 (I/O), MSD_D3RF3L_34 (I/O), MSD_D3RF3L_40 (I/O), MSD_D3RF3L_48 (I/O), MSD_D3RF3L_ODT120 (Input), MSD_D3RF3L_ODT40 (Input), MSD_D3RF3L_ODT60 (Input), MSD_D3RF3L_ODTOFF (Input), MSD_D3RF3_ODT120 (Input), MSD_D3RF3_ODT40 (Input), MSD_D3RF3_ODT60 (Input), MSD_D3RF3_ODTOFF (Input), MSD_D3RFL2_34 (I/O), MSD_D3RFL2_40 (I/O), MSD_D3RFL2_48 (I/O), MSD_D3RFL2_60 (I/O), MSD_D3RFL2_80 (I/O), MSD_D3RFL2_ODTOFF (Input), MSD_D3RFL_48 (I/O)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
